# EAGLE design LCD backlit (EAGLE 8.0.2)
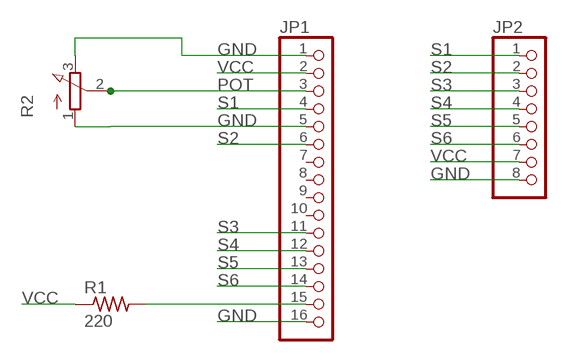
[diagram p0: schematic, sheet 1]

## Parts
JP1  PINHD-1X16  [1X16]
JP2  PINHD-1X8  [1X08]
R1  220  RES-US1206FAB  [R1206FAB]
R2  3RP/1610N  [3RP/1610N]

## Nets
GND: JP1.1 JP1.5 JP1.16 JP2.8 R2.1(A) R2.3(E)
N$1: JP1.15 R1.2
POT: JP1.3 R2.2(S)
S1: JP1.4 JP2.1
S2: JP1.6 JP2.2
S3: JP1.11 JP2.3
S4: JP1.12 JP2.4
S5: JP1.13 JP2.5
S6: JP1.14 JP2.6
VCC: JP1.2 JP2.7 R1.1
Unconnected: JP1.7 JP1.8 JP1.9 JP1.10

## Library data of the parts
JP1 = pinhead:PINHD-1X16: PIN HEADER
JP2 = pinhead:PINHD-1X8: PIN HEADER
R1 = fab:RES-US: Resistor (US Symbol)
R2 = pot:3RP/1610N: 16mm Potentiometer one level Source: http://www.alphapotentiometers.net/html/16mm_pot_2.html

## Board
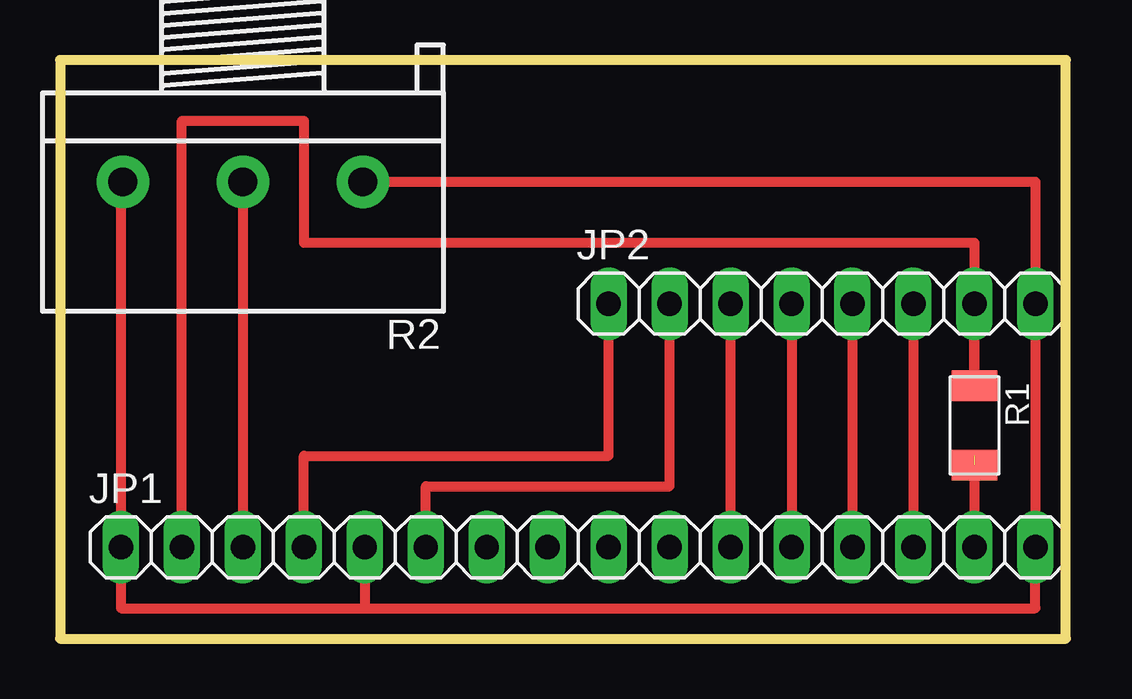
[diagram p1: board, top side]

Size 41.91 x 24.13 mm. Coordinates in mm from the lower left corner, seen from the top.
Outline: 0,0 41.91,0 41.91,24.13 0,24.13 0,0
Copper layers (1*16): Top 0.035mm / dielectric 1.5mm / Bottom 0.035mm
Design rules "default": minimum track width 10mil, minimum drill 24mil, track to track 8mil, track to pad 8mil, pad to pad 8mil, via to via 8mil, smd to smd 8mil, copper to edge 40mil, drill to drill 8mil, minimum pad ring 10mil, minimum via ring 8mil, stop-mask expansion 4mil, vias tented up to drill 0mil, thermal gap 10mil

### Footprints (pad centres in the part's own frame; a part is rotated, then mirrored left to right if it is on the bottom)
1X16 = drill 1.016 long: 1 -19.05,0; 2 -16.51,0; 3 -13.97,0; 4 -11.43,0; 5 -8.89,0; 6 -6.35,0; 7 -3.81,0; 8 -1.27,0; 9 1.27,0; 10 3.81,0; 11 6.35,0; 12 8.89,0; 13 11.43,0; 14 13.97,0; 15 16.51,0; 16 19.05,0
1X08 = drill 1.016 long: 1 -8.89,0; 2 -6.35,0; 3 -3.81,0; 4 -1.27,0; 5 1.27,0; 6 3.81,0; 7 6.35,0; 8 8.89,0
R1206FAB = smd 1.27 x 1.905: 1 -1.651,0; 2 1.651,0
3RP/1610N = drill 1.2 pad 2.184: 1 -5,0; 2 0,0; 3 5,0

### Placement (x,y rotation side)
JP1  21.59,3.81 0 top
JP2  31.75,13.97 0 top
R1  38.1,8.89 270 top
R2  7.62,19.05 180 top

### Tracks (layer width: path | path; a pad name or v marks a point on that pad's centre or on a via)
GND
  Top 0.406: 12.7,1.27 2.54,1.27 JP1.1 2.54,19.05 R2.3 | 12.7,1.27 40.64,1.27 JP1.16 JP2.8 40.64,19.05 R2.1 | JP1.5 12.7,1.27
N$1  (1 unrouted)
  Top 0.406: 38.1,7.62 JP1.15
POT
  Top 0.406: R2.2 JP1.3
S1
  Top 0.406: JP1.4 10.16,7.62 22.86,7.62 JP2.1
S2
  Top 0.406: JP1.6 15.24,6.35 25.4,6.35 JP2.2
S3
  Top 0.406: JP1.11 JP2.3
S4
  Top 0.406: JP2.4 JP1.12
S5
  Top 0.406: JP2.5 JP1.13
S6
  Top 0.406: JP2.6 JP1.14
VCC
  Top 0.406: R1.1 JP2.7 | R1.1 38.1,10.16 | R1.1 38.1,16.51 10.16,16.51 10.16,21.59 5.08,21.59 JP1.2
